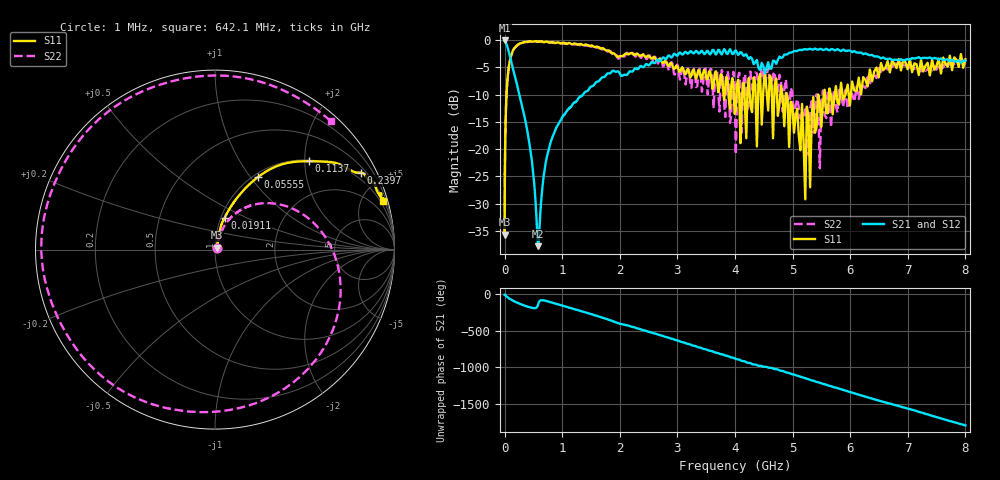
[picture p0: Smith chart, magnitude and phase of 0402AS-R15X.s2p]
!s-Parameter Generated by FASTRON Sdn. Bhd.
!FASTRON P/N : 0402AS-R15X
!Keysight Technologies: E5071C_MY46733604_B.14.02
!Date: Mon Dec 01 10:49:30 2025
!Version  :Rev00  Mon Dec 01 10:49:30 2025
!Data & Calibration Information:
!Freq  S11:SOLT2(ON)  S21:SOLT2(ON)  S12:SOLT2(ON)  S22:SOLT2(ON)
!PortZ  Port1:50+j0  Port2:50+j0
!When reading reference impedance value at option line is always used.
! Remarks : This data is being provided solely for informational purposes.
# Hz S dB R 50
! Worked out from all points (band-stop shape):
!   1601 points, 1 MHz to 8 GHz, reference 50 ohm
!   highest |S21| = -0.06 dB at 1.31 MHz (marker M1); lowest = -37.8 dB at 584.6 MHz (marker M2)
!   |S21| within 3 dB of the highest: 2.909 GHz to 4.216 GHz (1.307 GHz wide, 36.7 % of centre); 4.834 GHz to 6.491 GHz (1.657 GHz wide, 29.3 % of centre)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
!   lowest |S11| = -35.7 dB at 1.007 MHz (marker M3), VSWR 1.03, Z = 51.3 + j1.06 ohm
!   |S11| at or under -10 dB: 4.897 GHz to 5.444 GHz (547.5 MHz wide, 10.6 % of centre); 5.445 GHz to 5.544 GHz (98.93 MHz wide, 1.8 % of centre); 5.666 GHz to 5.731 GHz (64.99 MHz wide, 1.14 % of centre)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
!   |S22| runs from -35.7 to -0.2 dB; largest |S21 - S12| = 0.023
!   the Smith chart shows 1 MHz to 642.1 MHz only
!   S11 on the Smith chart (normalised r, x): 1 MHz: 1.03, +0.02; 19.11 MHz: 1.04, +0.38; 55.55 MHz: 1.05, +1.09; 113.7 MHz: 1.03, +2.10; 239.7 MHz: 0.73, +3.91; 642.1 MHz: 0.68, +7.01
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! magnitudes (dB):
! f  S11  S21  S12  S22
! 1 MHz  -35.4  -0.1  -0.1  -35.3
! 1.007 MHz  -35.7  -0.1  -0.1  -35.5
! 1.31 MHz  -34.3  -0.1  -0.1  -34.7
! 4.479 MHz  -26.6  -0.1  -0.1  -26.6
! 19.11 MHz  -14.6  -0.3  -0.3  -14.6
! 20.07 MHz  -14.2  -0.3  -0.3  -14.2
! 55.55 MHz  -6.6  -1.4  -1.4  -6.6
! 89.95 MHz  -3.9  -2.8  -2.8  -3.9
! 113.7 MHz  -2.9  -3.8  -3.8  -2.9
! 239.7 MHz  -0.8  -9.2  -9.2  -0.8
! 400.7 MHz  -0.3  -17.0  -17.0  -0.3
! 496.1 MHz  -0.3  -24.2  -24.1  -0.2
! 584.6 MHz  -0.3  -37.8  -37.7  -0.3
! 642.1 MHz  -0.2  -28.7  -28.7  -0.3
! 850.7 MHz  -0.4  -17.3  -17.3  -0.5
! 1.795 GHz  -1.9  -6.1  -6.1  -2.1
! 2.707 GHz  -3.6  -3.8  -3.8  -3.3
! 3.974 GHz  -8.5  -2.5  -2.5  -5.8
! 4.577 GHz  -12.9  -4.0  -4.1  -5.0
! 5.164 GHz  -11.7  -1.8  -1.9  -13.8
! 6.651 GHz  -3.8  -3.5  -3.5  -5.4
! 8 GHz  -3.5  -3.8  -3.8  -4.5
